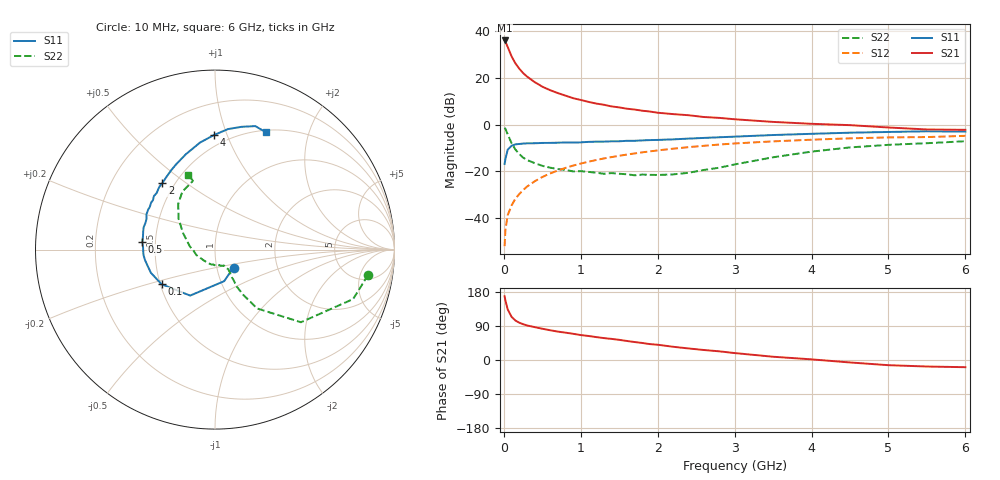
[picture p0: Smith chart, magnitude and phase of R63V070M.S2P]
! SIEMENS Small Signal Semiconductors
! BFR193
! Si NPN RF Bipolar Junction Transistor in SOT23
! VCE = 3 V  IC = 70 mA
! Common Emitter S-Parameters:  May  1996
# GHz  S  MA  R  50
!  f  S11  S21  S12  S22
! GHz  MAG  ANG  MAG  ANG  MAG  ANG  MAG  ANG
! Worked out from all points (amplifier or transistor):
!   36 points, 10 MHz to 6 GHz, reference 50 ohm
!   highest |S21| = 36.1 dB at 10 MHz (marker M1)
!   |S21| within 3 dB of that: start of sweep to 52.75 MHz
!   unconditionally stable (mu >= 1): 292.5 MHz to 1.889 GHz; 1.908 GHz to 2.122 GHz
!   at 250 MHz: K = 0.99, MSG = 25.1 dB, |S12| = -28.0 dB
!   at 1.4 GHz: K = 1.02, MAG = 9.9 dB, |S12| = -13.9 dB
!   at 6 GHz: K = 0.97, MSG = 1.3 dB, |S12| = -4.8 dB
!   S11 on the Smith chart (normalised r, x): 10 MHz: 1.20, -0.25; 100 MHz: 0.51, -0.22; 500 MHz: 0.42, +0.04; 2 GHz: 0.43, +0.41; 4 GHz: 0.42, +0.90; 6 GHz: 0.52, +1.39
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0.01  0.1442 -44.1  63.99 168.3  0.0025 81.0  0.8644 -9.4
0.02  0.1832 -73.9  60.57 157.5  0.0055 76.2  0.8175 -19.7
0.05  0.2913 -118.4  46.46 133.6  0.0115 71.4  0.627 -40.2
0.1  0.3546 -147.0  29.34 114.1  0.0186 70.2  0.4033 -54.4
0.15  0.3799 -160.1  20.75 104.2  0.026 73.9  0.2952 -58.1
0.2  0.3872 -167.2  15.95 98.5  0.0326 74.2  0.2361 -59.6
0.25  0.3944 -171.6  12.84 94.5  0.0397 75.0  0.1977 -58.6
0.3  0.3998 -175.9  10.82 91.2  0.0471 76.2  0.1758 -58.9
0.4  0.401 178.4  8.212 86.8  0.0613 75.9  0.1508 -56.8
0.5  0.4074 173.9  6.55 82.5  0.0758 75.6  0.1316 -56.0
0.6  0.4083 169.3  5.517 78.6  0.0901 74.4  0.1204 -58.2
0.7  0.4122 166.1  4.778 75.0  0.1044 73.2  0.1123 -59.4
0.9  0.4152 158.5  3.711 69.2  0.1332 70.9  0.1001 -61.0
1.1  0.4294 152.8  3.088 63.4  0.1614 68.1  0.0976 -67.0
1.4  0.442 143.7  2.469 55.7  0.2027 63.7  0.0921 -80.0
2  0.4727 128.4  1.808 40.3  0.2818 54.3  0.0839 -118.9
2.2  0.4858 124.1  1.69 34.9  0.3067 51.1  0.0863 -134.0
3.5  0.602 98.0  1.15 8.6  0.4404 30.1  0.2007 152.6
4  0.639 90.4  1.047 1.7  0.4777 23.0  0.2655 139.8
4.5  0.6756 83.8  0.98 -6.5  0.5112 15.8  0.3266 128.9
5.5  0.7238 71.9  0.792 -17.2  0.5443 2.1  0.4021 107.8
6  0.7125 66.7  0.778 -19.0  0.5781 -2.0  0.4436 109.7
